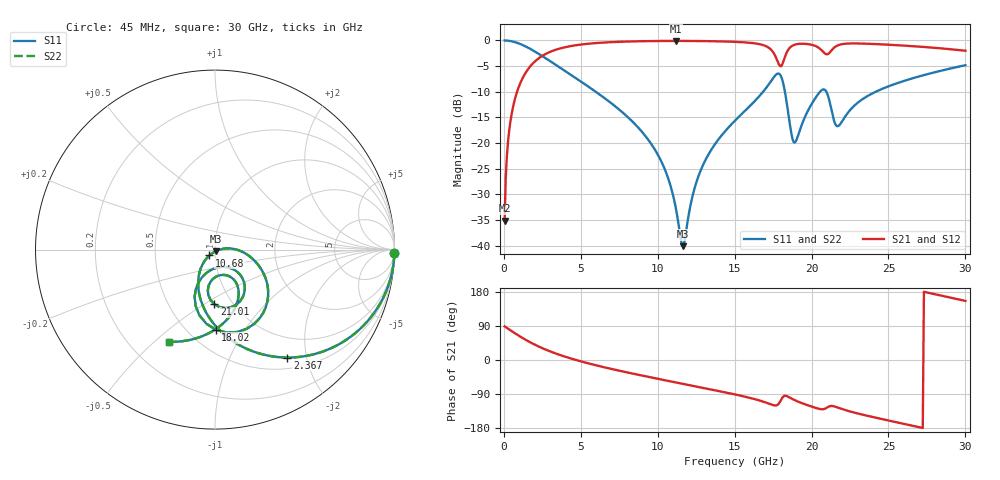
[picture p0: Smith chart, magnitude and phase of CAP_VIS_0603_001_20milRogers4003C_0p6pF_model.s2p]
! S-parameter model data by Modelithics Inc.  support@modelithics.com  813-866-6335  Tampa FL USA
! S-Parameter data specifications:
! Substrate: 20-mil Rogers 4003C, substrate thickness, H=0.508mm, Dielectric constant, Er=3.75
! PCB Mounting Pad Footprint: Pad width, PadW=0.90mm , Pad length, PadL=1.00mm , Pad gap, PadG (edge-to-edge)=1.00mm , Reference planes=3.0mm apart
! Created Wed Nov 18 13:16:38 2015
# hz S ma R 50
! 2 Port Network Data from SP1.SP block
! freq  magS11  angS11  magS21  angS21  magS12  angS12  magS22  angS22
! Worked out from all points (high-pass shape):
!   401 points, 45 MHz to 30 GHz, reference 50 ohm
!   highest |S21| = -0.09 dB at 11.2 GHz (marker M1); lowest = -35.2 dB at 45 MHz (marker M2)
!   |S21| within 3 dB of the highest: 2.451 GHz to 17.65 GHz (15.2 GHz wide, 151 % of centre); 18.28 GHz to end of sweep
!   lowest |S11| = -40.1 dB at 11.65 GHz (marker M3), VSWR 1.02, Z = 50.5 - j0.85 ohm
!   |S11| at or under -10 dB: 5.966 GHz to 16.85 GHz (10.88 GHz wide, 95.4 % of centre); 18.27 GHz to 20.55 GHz (2.285 GHz wide, 11.8 % of centre); 20.96 GHz to 24.18 GHz (3.216 GHz wide, 14.2 % of centre)
!   |S22| runs from -40.1 to 0.0 dB; largest |S21 - S12| = 0
!   S11 on the Smith chart (normalised r, x): 45 MHz: 1, -92; 2.367 GHz: 0.66, -1.67; 10.68 GHz: 0.94, -0.06; 18.02 GHz: 0.67, -0.75; 21.01 GHz: 0.83, -0.55; 30 GHz: 0.37, -0.56
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4.5e7  0.9998 -1.2  0.01745 88.8  0.01745 88.8  0.9998 -1.2
3.4455e8  0.9911 -9.5  0.1326 80.5  0.1326 80.5  0.9911 -9.5
7.189875e8  0.9628 -19.5  0.2693 70.5  0.2693 70.5  0.9628 -19.5
1.392975e9  0.8768 -36.2  0.4792 53.7  0.4792 53.7  0.8768 -36.2
2.366512e9  0.7238 -56.2  0.687 33.6  0.687 33.6  0.7238 -56.2
5.062462e9  0.3921 -93.5  0.9142 -4.2  0.9142 -4.2  0.3921 -93.5
8.282625e9  0.1658 -122.6  0.978 -35.1  0.978 -35.1  0.1658 -122.6
1.007992e10  0.07333 -133.4  0.9878 -50.2  0.9878 -50.2  0.07333 -133.4
1.067902e10  0.04521 -133.5  0.989 -55.1  0.989 -55.1  0.04521 -133.5
1.120324e10  0.02203 -123.9  0.9893 -59.3  0.9893 -59.3  0.02203 -123.9
1.165256e10  0.009856 -58.6  0.9891 -62.9  0.9891 -62.9  0.009856 -58.6
1.285076e10  0.05669 6.1  0.9862 -72.6  0.9862 -72.6  0.05669 6.1
1.50225e10  0.1652 -6.4  0.969 -90.8  0.969 -90.8  0.1652 -6.4
1.734401e10  0.3969 -41.9  0.819 -116.9  0.819 -116.9  0.3969 -41.9
1.8018e10  0.4464 -89.4  0.5611 -105.0  0.5611 -105.0  0.4464 -89.4
1.831755e10  0.2858 -113.4  0.7235 -94.5  0.7235 -94.5  0.2858 -113.4
1.884176e10  0.1018 -85.6  0.9015 -104.7  0.9015 -104.7  0.1018 -85.6
2.003996e10  0.2447 -48.6  0.9054 -123.3  0.9054 -123.3  0.2447 -48.6
2.10135e10  0.3048 -90.5  0.7323 -125.3  0.7323 -125.3  0.3048 -90.5
2.168749e10  0.1455 -78.2  0.8931 -125.3  0.8931 -125.3  0.1455 -78.2
2.505742e10  0.3596 -73.8  0.9078 -160.2  0.9078 -160.2  0.3596 -73.8
3e10  0.5736 -116.3  0.7935 155.9  0.7935 155.9  0.5736 -116.3
